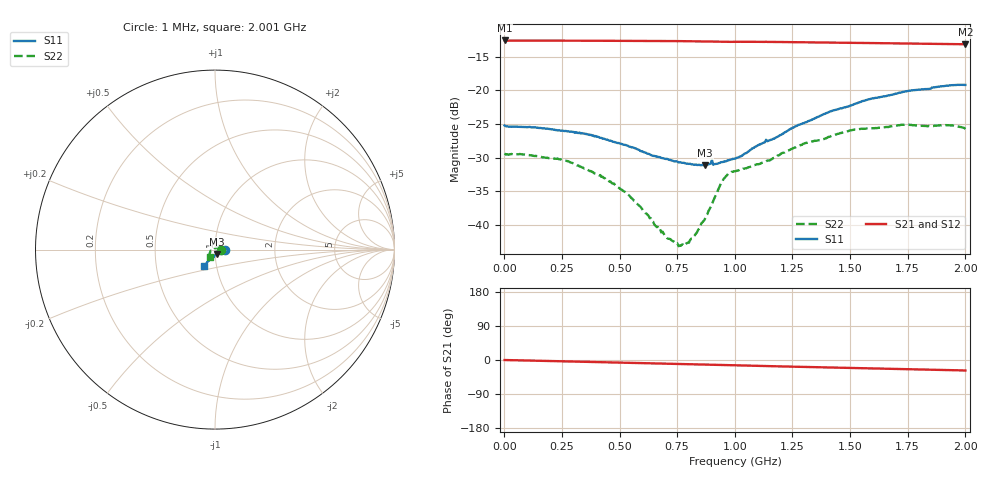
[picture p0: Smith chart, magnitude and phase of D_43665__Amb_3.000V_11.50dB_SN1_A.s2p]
! device id: 43665_
! dir: \\malibu\benchdata\1_engineers\tn_data\43665_75ohm\new\sparar\43665_\amb\3p000v\11p50db
! Serial: 1
! Insertion: A
! Temp: Amb
! VDD: 3.000V
! Attenuation Step: 11.50dB
! IDD: 1.452549e+00mA
! FILE NAME
! DATE 03-27-2009 08:36:11
! CORRECTED  DATA
#  Hz  S  RI  R  75
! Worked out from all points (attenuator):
!   401 points, 1 MHz to 2.001 GHz, reference 75 ohm
!   highest |S21| = -12.57 dB at 1 MHz (marker M1); lowest = -13.1 dB at 2.001 GHz (marker M2)
!   lowest |S11| = -31.1 dB at 871 MHz (marker M3), VSWR 1.06, Z = 76.7 - j3.84 ohm
!   |S11| at or under -10 dB: start of sweep to end of sweep
!   |S22| runs from -43.2 to -25.1 dB; largest |S21 - S12| = 0.00071
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1000000  0.0548 -0.000823  0.2352 -0.000393  0.2352 -0.000478  0.034 -0.000316
2.36e8  0.0504 -0.00341  0.2341 -0.0131  0.2341 -0.0132  0.0295 0.009
3.36e8  0.0479 -0.00555  0.2335 -0.0187  0.2335 -0.0188  0.0242 0.0116
4.26e8  0.0433 -0.00724  0.2328 -0.0237  0.2329 -0.0239  0.0193 0.0123
5.31e8  0.0374 -0.0108  0.2316 -0.0299  0.2317 -0.03  0.0127 0.0115
6.26e8  0.0308 -0.0139  0.2304 -0.0349  0.2304 -0.0352  0.00517 0.0105
6.71e8  0.0278 -0.0159  0.2299 -0.0375  0.2299 -0.0378  0.00287 0.00873
7.06e8  0.0256 -0.0174  0.2295 -0.0396  0.2295 -0.0398  0.000589 0.00798
7.71e8  0.0207 -0.0202  0.2284 -0.0434  0.2284 -0.0436  -0.00429 0.00573
7.91e8  0.0192 -0.0211  0.228 -0.0446  0.2281 -0.0449  -0.00584 0.00441
8.26e8  0.0162 -0.0228  0.2274 -0.0467  0.2274 -0.047  -0.0082 0.00161
8.71e8  0.0121 -0.025  0.2263 -0.0495  0.2262 -0.0497  -0.0109 -0.00237
9.51e8  0.00558 -0.0289  0.2235 -0.0536  0.2236 -0.0534  -0.0208 -0.00698
9.76e8  0.0038 -0.0301  0.2231 -0.0543  0.2232 -0.0541  -0.0234 -0.00619
1.001e9  0.00157 -0.0311  0.223 -0.0554  0.2231 -0.0553  -0.0244 -0.00576
1.146e9  -0.0108 -0.0408  0.2204 -0.0637  0.2206 -0.0635  -0.0266 -0.0142
1.336e9  -0.0275 -0.0542  0.2155 -0.0735  0.2158 -0.0733  -0.032 -0.0269
1.511e9  -0.0406 -0.0668  0.2102 -0.0821  0.2106 -0.0822  -0.0349 -0.037
1.671e9  -0.0495 -0.0777  0.2054 -0.0894  0.2056 -0.0896  -0.0342 -0.0414
1.731e9  -0.0527 -0.082  0.2035 -0.092  0.2039 -0.0922  -0.0338 -0.044
1.921e9  -0.0597 -0.0906  0.1977 -0.0993  0.1978 -0.0994  -0.0328 -0.0443
2.001e9  -0.0601 -0.0919  0.1953 -0.1022  0.1948 -0.1028  -0.0298 -0.0424
